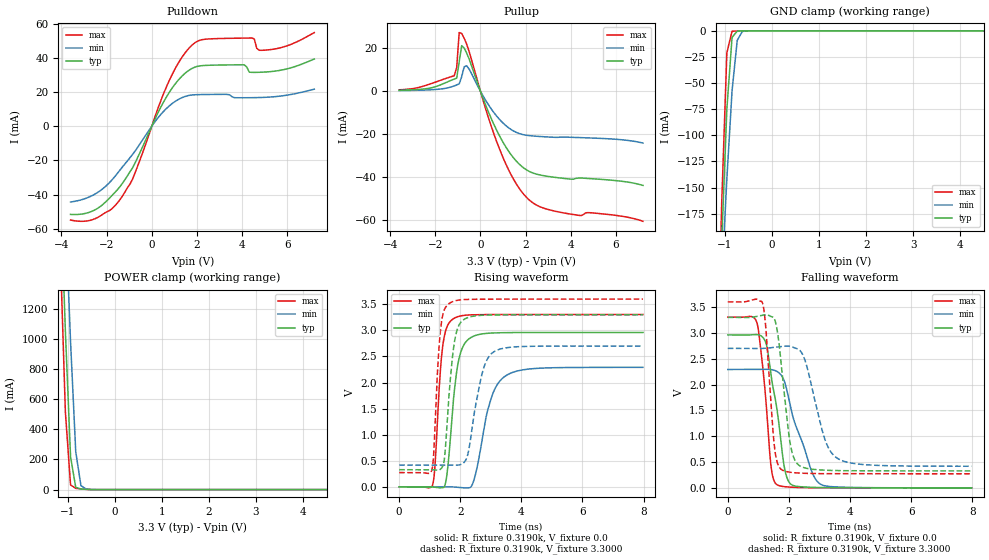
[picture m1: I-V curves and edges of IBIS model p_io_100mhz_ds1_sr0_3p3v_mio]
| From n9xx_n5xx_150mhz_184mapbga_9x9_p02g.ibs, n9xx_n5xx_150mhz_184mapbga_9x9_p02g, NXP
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[Model] p_io_100mhz_ds1_sr0_3p3v_mio
|   Model p_io_100mhz_ds1_sr0_3p3v_mio
| This model was characterised for following simulation conditions:
| External (pad) voltage:
|   - Typ: 3.3V,   - Min: 2.7V,   - Max: 3.6V
| Library cells for typ/min/max conditions are connected as defined below:
|  pad - External Pad
|  ipp_do_lv - Core Input
|  ipp_obe_lv - Output Buffer Enable
|  IOGC - NC
|  REFH3V3 - REFH3V3
|  REFL3V3 - REFL3V3
|  ZI - NC
|  abut_ncal_vddio[1] - vddio
|  abut_ncal_vddio[2] - vddio
|  abut_ncal_vddio[3] - vssio
|  abut_ncal_vddio[4] - vddio
|  abut_ncal_vddio[5] - vddio
|  abut_ncal_vddio[6] - vssio
|  abut_pcal_vddio[1] - vssio
|  abut_pcal_vddio[2] - vssio
|  abut_pcal_vddio[3] - vddio
|  abut_pcal_vddio[4] - vssio
|  abut_pcal_vddio[5] - vssio
|  abut_pcal_vddio[6] - vddio
|  ipp_do_1p8v - ipp_do_1p8v
|  ipp_dse_lv - vdd_lv
|  ipp_eftd_lv - NC
|  ipp_ina_mux_vddio - NC
|  ipp_ina_mux_vddio[0] - NC
|  ipp_ina_mux_vddio[1] - NC
|  ipp_ina_r0_vddio - NC
|  ipp_ina_r0a_vddio - NC
|  ipp_ina_r0b_vddio - NC
|  ipp_ina_r0c_vddio - NC
|  ipp_ina_r0d_vddio - NC
|  ipp_ina_r0e_vddio - NC
|  ipp_ina_r0f_vddio - NC
|  ipp_ina_r300_vddio - NC
|  ipp_ina_r300a_vddio - NC
|  ipp_ina_r300b_vddio - NC
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Model_type I/O
Polarity   Non-Inverting
Enable   Active-High
Vinl =   0.9900V
Vinh =   2.3100V
Vmeas =  1.6500V
Cref =   30.0000pF
Rref =   1.0000M
Vref =   3.3000V
C_comp   1.3235pF   1.2640pF   1.4076pF
|C_comp_pullup   0.6739pF   0.7056pF   0.6519pF
|C_comp_pulldown   0.5816pF   0.6344pF   0.5434pF
[Model Spec]
| variable   typ   min   max
Vinh   2.3100V   1.8900V   2.5200V
Vinl   0.9900V   0.8100V   1.0800V
[Temperature Range]   25.0000   0.1250k   -40.0000
[Voltage Range]   3.3000V   2.7000V   3.6000V
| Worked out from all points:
|   slope of the pulldown table from 0 to 0.495 V, typ, clamps not added: 36.6 ohm
|   slope of the pullup table from 0 to 0.495 V, typ, clamps not added: 37.7 ohm
|   GND clamp passes 1 mA (typ) near -0.75 V on its own axis
|   POWER clamp passes 1 mA (typ) near -0.55 V on its own axis
|   rising waveform, R_fixture 0.3190k, V_fixture 0.0: 20-80 % time 299ps typ, 517ps min, 214ps max; typ from 0 V to 2.96 V
|   rising waveform, R_fixture 0.3190k, V_fixture 3.3000: 20-80 % time 255ps typ, 423ps min, 184ps max; typ from 0.328 V to 3.3 V
|   falling waveform, R_fixture 0.3190k, V_fixture 0.0: 20-80 % time 427ps typ, 707ps min, 290ps max; typ from 2.96 V to 0 V
|   falling waveform, R_fixture 0.3190k, V_fixture 3.3000: 20-80 % time 330ps typ, 583ps min, 237ps max; typ from 3.3 V to 0.329 V
[Pulldown]
|Voltage   I(typ)   I(min)   I(max)
-3.6V     -51.52mA   -44.27mA   -54.81mA
-2.5V     -48.75mA   -39.51mA   -53.96mA
-1.4V     -35.12mA   -25.45mA   -42.73mA
-850mV    -24.27mA   -16.41mA   -30.84mA
800mV     20.29mA    12.16mA    27.43mA
1.35V     29.44mA    16.78mA    40.57mA
1.9V      34.5mA     18.39mA    48.67mA
4.1V      35.87mA    16.66mA    51.51mA
4.43V     31.5mA     16.69mA    51.59mA
4.65V     31.5mA     16.75mA    45.53mA
5.09V     31.75mA    16.96mA    44.55mA
7.2V      39.3mA     21.67mA    54.74mA
[Pullup]
|Voltage   I(typ)   I(min)   I(max)
-3.6V     391.8uA    234.9uA    605.7uA
-1.16V    5.604mA    2.419mA    7.14mA
-1.05V    6.055mA    2.871mA    11mA
-940mV    13.56mA    3.339mA    27.24mA
-830mV    21.15mA    6.685mA    26.82mA
-720mV    20.05mA    11.26mA    24.61mA
-610mV    17.74mA    11.81mA    21.86mA
820mV     -20.29mA   -12.86mA   -26.23mA
1.48V     -31.23mA   -18.63mA   -41.23mA
2.03V     -36.57mA   -20.53mA   -49.31mA
3.46V     -40.33mA   -21.49mA   -56.22mA
7.2V      -43.87mA   -24.17mA   -60.58mA
[GND_clamp]
|Voltage   I(typ)   I(min)   I(max)
-3.6V     -4.134A    -3.035A    -5.609A
-1.18V    -349.4mA   -343.6mA   -365.7mA
-1.07V    -202.9mA   -239.3mA   -165.2mA
-960mV    -74.83mA   -141.5mA   -21.03mA
-850mV    -6.389mA   -57.64mA   -383.3uA
-740mV    -222.1uA   -9.174mA   -124.1uA
-630mV    -55.93uA   -558.9uA   -58.07uA
7.2V      0A         0A         0A
[POWER_clamp]
|Voltage   I(typ)   I(min)   I(max)
-3.6V     24.54A     22.33A     26.93A
-1.16V    2.046A     2.721A     1.599A
-1.05V    1.052A     1.847A     514.4mA
-940mV    218.6mA    981.8mA    31.16mA
-830mV    15.1mA     252.4mA    8.462mA
-720mV    4.281mA    26.81mA    4.453mA
-610mV    1.717mA    3.626mA    1.66mA
7.2V      0A         0A         0A
[Ramp]
| variable   typ   min   max
dV/dt_r  1.7763/0.2988n   1.3750/0.5172n   1.9832/0.2140n
dV/dt_f  1.7828/0.3303n   1.3691/0.5828n   1.9962/0.2366n
R_load = 0.3190k
[Rising Waveform]
R_fixture= 0.3190k
V_fixture= 0.0
V_fixture_min= 0.0
V_fixture_max= 0.0
|time   V(typ)   V(min)   V(max)
0s        2.902nV    250nV      9.459nV
1.087ns   -979.7uV   -29.68uV   18.97mV
1.414ns   -15.49mV   651.6uV    2.638V
1.568ns   248.6mV    1.45mV     3.071V
1.765ns   1.587V     -2.092mV   3.22V
2.173ns   2.773V     -19.8mV    3.292V
2.455ns   2.894V     144.3mV    3.3V
3.051ns   2.95V      1.762V     3.304V
3.489ns   2.957V     2.13V      3.305V
7.98ns    2.961V     2.292V     3.305V
[Rising Waveform]
R_fixture= 0.3190k
V_fixture= 3.3000
V_fixture_min= 2.7000
V_fixture_max= 3.6000
|time   V(typ)   V(min)   V(max)
0s        328.4mV    417.4mV    273mV
1.073ns   327.9mV    417.3mV    324.5mV
1.355ns   338.7mV    417.7mV    3.015V
1.483ns   540.3mV    418.3mV    3.4V
1.64ns    1.82V      417.6mV    3.518V
1.968ns   3.111V     420.4mV    3.583V
2.25ns    3.247V     626mV      3.595V
2.767ns   3.292V     2.277V     3.599V
3.119ns   3.297V     2.597V     3.6V
7.98ns    3.3V       2.7V       3.6V
[Falling Waveform]
R_fixture= 0.3190k
V_fixture= 0.0
V_fixture_min= 0.0
V_fixture_max= 0.0
|time   V(typ)   V(min)   V(max)
0s        2.961V     2.292V     3.305V
962.1ps   2.966V     2.29V      3.18V
1.243ns   2.814V     2.294V     1.729V
1.42ns    2.165V     2.29V      401.7mV
1.604ns   1.547V     2.256V     63.32mV
1.828ns   484.5mV    2.1V       25.21mV
1.983ns   134.2mV    1.765V     16.47mV
2.726ns   10.64mV    351.6mV    2.554mV
3.028ns   5.806mV    73.86mV    1.287mV
7.98ns    91.01uV    217.7uV    57.56uV
[Falling Waveform]
R_fixture= 0.3190k
V_fixture= 3.3000
V_fixture_min= 2.7000
V_fixture_max= 3.6000
|time   V(typ)   V(min)   V(max)
0s        3.3V       2.7V       3.6V
1.141ns   3.342V     2.699V     3.572V
1.245ns   3.351V     2.703V     3.1V
1.521ns   3.275V     2.72V      833.3mV
1.761ns   2.328V     2.737V     352.6mV
2.062ns   799.5mV    2.736V     300.5mV
2.38ns    418.5mV    2.648V     284.7mV
3.171ns   341.9mV    952.2mV    274.9mV
3.587ns   334.4mV    572.5mV    273.9mV
7.98ns    328.6mV    418.2mV    273.1mV
